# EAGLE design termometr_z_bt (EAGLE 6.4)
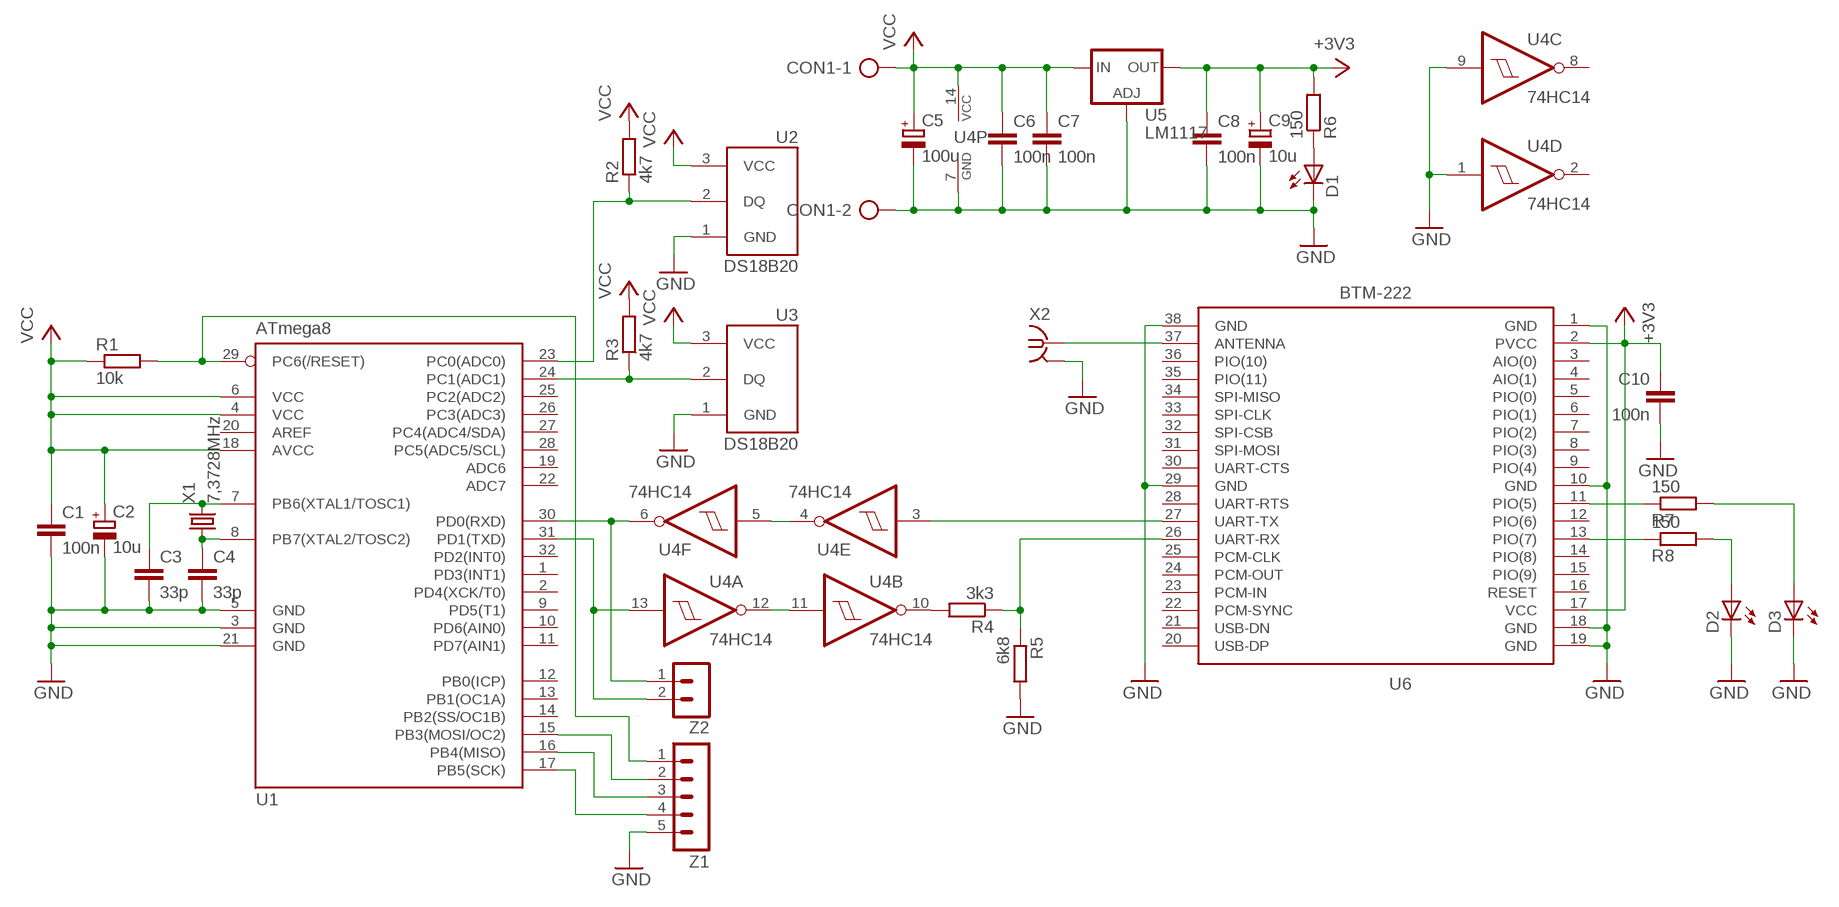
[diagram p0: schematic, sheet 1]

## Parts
C1  100n  C-EUC1206  [C1206]
C2  10u  CPOL-EUE2.5-5  [E2,5-5]
C3  33p  C-EUC1206  [C1206]
C4  33p  C-EUC1206  [C1206]
C5  100u  CPOL-EUE2.5-5  [E2,5-5]
C6  100n  C-EUC1206  [C1206]
C7  100n  C-EUC1206  [C1206]
C8  100n  C-EUC1206  [C1206]
C9  10u  CPOL-EUE2.5-5  [E2,5-5]
C10  100n  C-EUC1206  [C1206]
CON1  AK500/2  [AK500/2]
D1  LED5MM  [LED5MM]
D2  LED5MM  [LED5MM]
D3  LED5MM  [LED5MM]
R1  10k  R-EU_R1206  [R1206]
R2  4k7  R-EU_R1206  [R1206]
R3  4k7  R-EU_R1206  [R1206]
R4  3k3  R-EU_R1206  [R1206]
R5  6k8  R-EU_R1206  [R1206]
R6  150  R-EU_R1206  [R1206]
R7  150  R-EU_R1206  [R1206]
R8  150  R-EU_R1206  [R1206]
U1  ATmega8  MEGA8-AI  [TQFP32-08]
U2  DS18B20  [TO92-]
U3  DS18B20  [TO92-]
U4  74HC14  74HC14D  [SO14]
U5  LM1117  LD117AS50TR  [SOT223]
U6  BTM-222  BTM-222_ALL  [BTM-222]
X1  7,3728MHz  CRYSTALHC49S  [HC49/S]
X2  BU-SMA-G  [BU-SMA-G]
Z1  MA05-1  [MA05-1]
Z2  MA02-1  [MA02-1]

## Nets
+3V3: C8.1 C9.+ C10.1 R6.2 U5.4(OUT) U6.2(PVCC) U6.17(VCC)
GND: C1.2 C2.- C3.2 C4.2 C5.- C6.2 C7.2 C8.2 C9.- C10.2 CON1.2 D1.K(C) D2.K(C) D3.K(C) R5.2 U1.3(GND) U1.5(GND) U1.21(GND) U2.1(GND) U3.1(GND) U4.1(D:I) U4.7(P:GND) U4.9(C:I) U5.1(ADJ) U6.1(GND) U6.10(GND) U6.18(GND) U6.19(GND) U6.29(GND) U6.38(GND) X2.2(GND) Z1.5
N$1: D2.A R8.2
N$2: R7.1 U6.11(PIO(5))
N$3: D1.A R6.1
N$4: U4.3(E:I) U6.27(UART-TX)
N$5: R8.1 U6.13(PIO(7))
N$6: R1.2 U1.29(PC6(/RESET)) Z1.1
N$7: R2.1 U1.23(PC0(ADC0)) U2.2(DQ)
N$8: R3.1 U1.24(PC1(ADC1)) U3.2(DQ)
N$9: U4.11(B:I) U4.12(A:O)
N$10: U6.37(ANTENNA) X2.1
N$11: U4.4(E:O) U4.5(F:I)
N$12: U1.30(PD0(RXD)) U4.6(F:O) Z2.1
N$13: U1.31(PD1(TXD)) U4.13(A:I) Z2.2
N$14: R4.2 U4.10(B:O)
N$15: R4.1 R5.1 U6.26(UART-RX)
N$16: U1.15(PB3(MOSI/OC2)) Z1.2
N$17: U1.16(PB4(MISO)) Z1.3
N$18: U1.17(PB5(SCK)) Z1.4
N$19: D3.A R7.2
N$33: C3.1 U1.7(PB6(XTAL1/TOSC1)) X1.2
N$34: C4.1 U1.8(PB7(XTAL2/TOSC2)) X1.1
VCC: C1.1 C2.+ C5.+ C6.1 C7.1 CON1.1 R1.1 R2.2 R3.2 U1.4(VCC) U1.6(VCC) U1.18(AVCC) U2.3(VCC) U3.3(VCC) U4.14(P:VCC) U5.3(IN)
Unconnected: U1.1(PD3(INT1)) U1.2(PD4(XCK/T0)) U1.9(PD5(T1)) U1.10(PD6(AIN0)) U1.11(PD7(AIN1)) U1.12(PB0(ICP)) U1.13(PB1(OC1A)) U1.14(PB2(SS/OC1B)) U1.19(ADC6) U1.20(AREF) U1.22(ADC7) U1.25(PC2(ADC2)) U1.26(PC3(ADC3)) U1.27(PC4(ADC4/SDA)) U1.28(PC5(ADC5/SCL)) U1.32(PD2(INT0)) U4.2(D:O) U4.8(C:O) U6.3(AIO(0)) U6.4(AIO(1)) U6.5(PIO(0)) U6.6(PIO(1)) U6.7(PIO(2)) U6.8(PIO(3)) U6.9(PIO(4)) U6.12(PIO(6)) U6.14(PIO(8)) U6.15(PIO(9)) U6.16(RESET) U6.20(USB-DP) U6.21(USB-DN) U6.22(PCM-SYNC) U6.23(PCM-IN) U6.24(PCM-OUT) U6.25(PCM-CLK) U6.28(UART-RTS) U6.30(UART-CTS) U6.31(SPI-MOSI) U6.32(SPI-CSB) U6.33(SPI-CLK) U6.34(SPI-MISO) U6.35(PIO(11)) U6.36(PIO(10))

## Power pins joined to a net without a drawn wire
GND: X2.3(GND) X2.4(GND) X2.5(GND)

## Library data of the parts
C1 C3 C4 C6-C8 C10 = rcl:C-EU: CAPACITOR, European symbol
C2 C5 C9 = rcl:CPOL-EU: POLARIZED CAPACITOR, European symbol
CON1 = con-ptr500:AK500/2: CONNECTOR
D1-D3 = led:LED: LED
R1-R8 = rcl:R-EU_: RESISTOR, European symbol
U1 = atmel:MEGA8: MICROCONTROLLER 8 Kbytes FLASH, 1 kbytes SRAM, 512 bytes EEPROM, USART, 6-channel 10 bit ADC, 2-channel 8 bit ADC Pin compatible with Atmega48, ATMega88, ATMega168 Source: avr.lbr
U2 U3 = 1wire:DS18B20: Programmable Resolution Digital Thermometer This chip provides a onewire thermosensor with approx. 0.5°C accuracy. A programmable over/undertemperure alarm is available. The precision can be set from 9..12 bits. Notes: Vdd must be applied for accurate measurements at low temperatures, as the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
U4 = 74xx-eu:74*14: Hex schmitt trigger INVERTER
U5 = v-reg:LD117A?*: Low drop fixed and adjustable positive voltage regulators 1 A Source: http://www.st.com/stonline/products/literature/ds/7194/ld1117axx.pdf
U6 = bluetooth:BTM-222_ALL
X1 = crystal:CRYSTAL: CRYSTAL
X2 = con-coax:BU-SMA-G: FEMALE SMA CONNECTOR Radiall distributor RS 193-9117
Z1 = con-lstb:MA05-1: PIN HEADER
Z2 = con-lstb:MA02-1: PIN HEADER

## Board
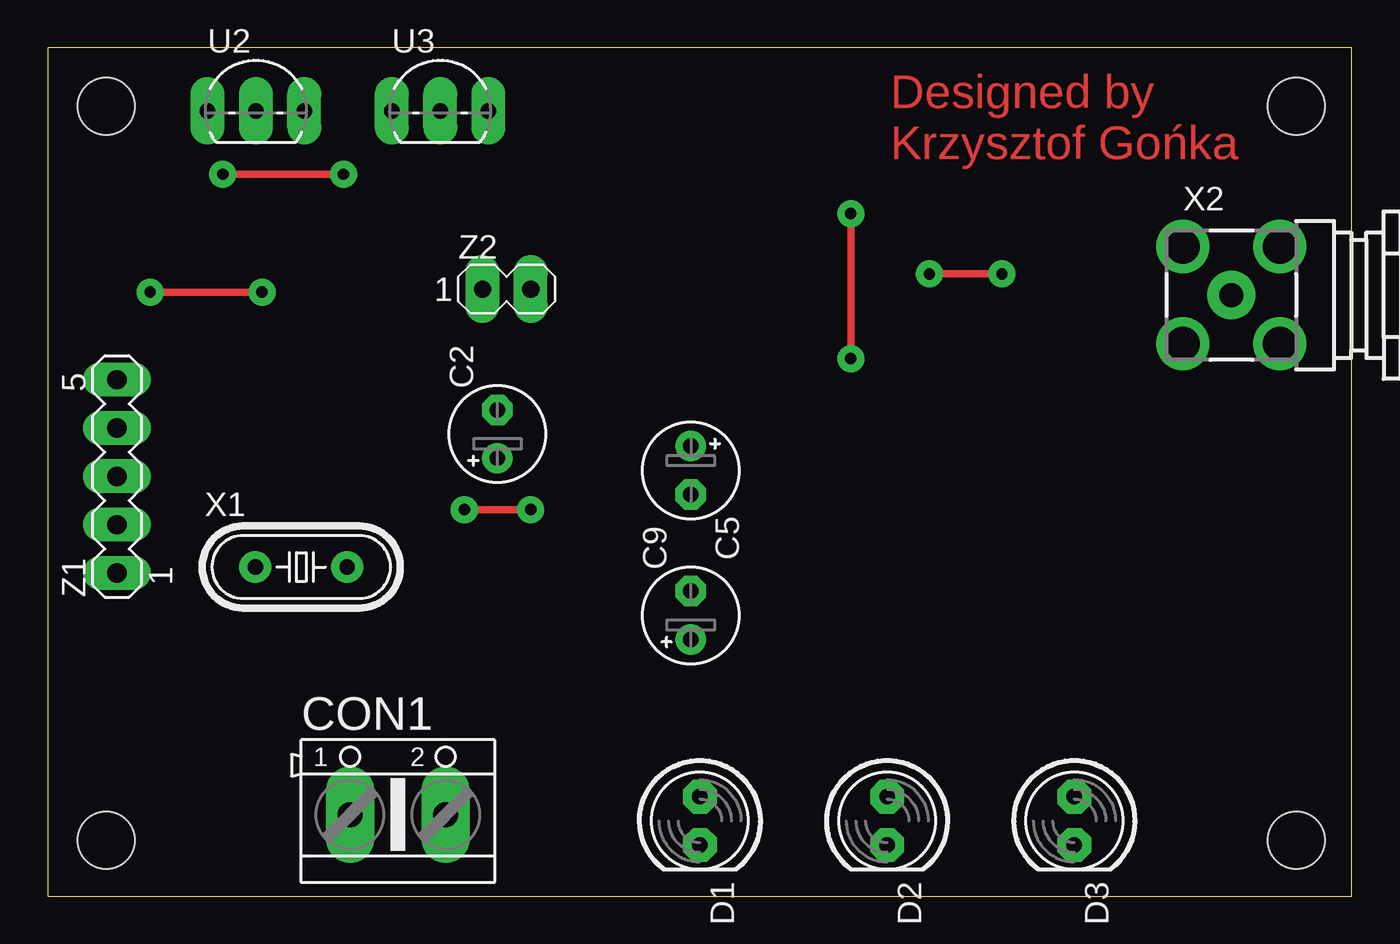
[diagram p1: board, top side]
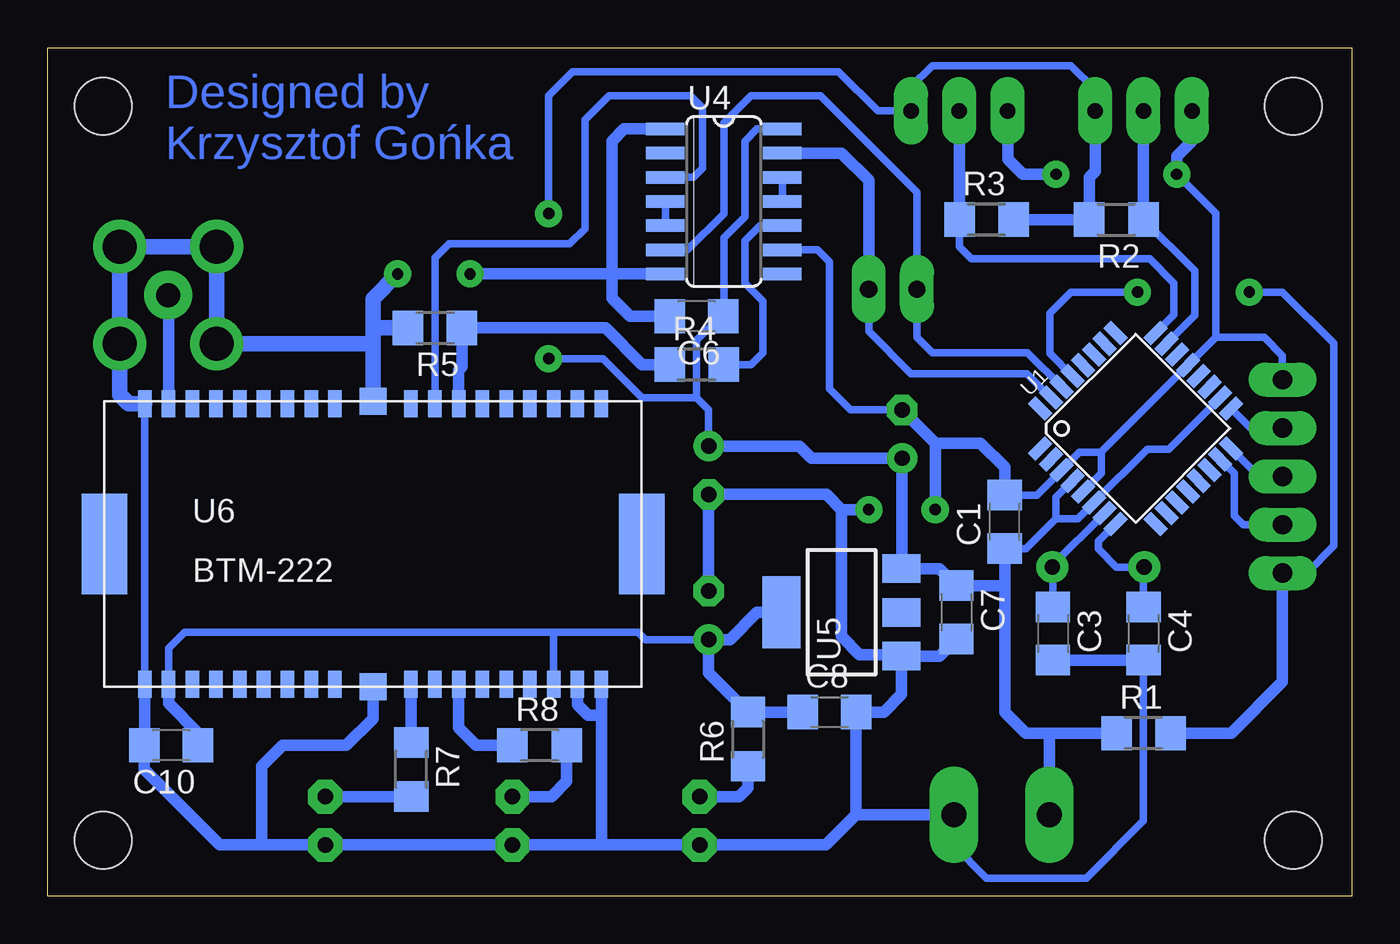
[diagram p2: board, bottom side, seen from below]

Size 68.57 x 44.6 mm. Coordinates in mm from the lower left corner, seen from the top.
Outline: 0,0 68.57,0 68.57,44.6 0,44.6 0,0
Copper layers (1*16): Top 0.035mm / dielectric 1.5mm / Bottom 0.035mm
Design rules "default": minimum track width 10mil, minimum drill 24mil, track to track 8mil, track to pad 8mil, pad to pad 8mil, via to via 8mil, smd to smd 8mil, copper to edge 40mil, drill to drill 8mil, minimum pad ring 10mil, minimum via ring 8mil, stop-mask expansion 4mil, vias tented up to drill 0mil, thermal gap 10mil
Holes 3 mm at 3.09,41.52 3.09,2.94 65.63,2.94 65.63,41.52

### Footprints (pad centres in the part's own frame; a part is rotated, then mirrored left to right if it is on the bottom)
C1206 = smd 1.6 x 1.8: 1 -1.4,0; 2 1.4,0
E2,5-5 = drill 0.813 pad 1.6: + -1.27,0 | drill 0.813 pad 1.6 octagon: - 1.27,0
AK500/2 = drill 1.321 pad 2.54 long: 1 -2.515,0; 2 2.515,0
LED5MM = drill 0.813 pad 1.778 octagon: A -1.27,0; K 1.27,0
R1206 = smd 1.6 x 1.803: 1 -1.422,0; 2 1.422,0
TQFP32-08 = smd 1.27 x 0.559: 1 -4.293,2.8; 2 -4.293,2; 3 -4.293,1.2; 4 -4.293,0.4; 5 -4.293,-0.4; 6 -4.293,-1.2; 7 -4.293,-2; 8 -4.293,-2.8; 17 4.293,-2.8; 18 4.293,-2; 19 4.293,-1.2; 20 4.293,-0.4; 21 4.293,0.4; 22 4.293,1.2; 23 4.293,2; 24 4.293,2.8 | smd 0.559 x 1.27: 9 -2.8,-4.293; 10 -2,-4.293; 11 -1.2,-4.293; 12 -0.4,-4.293; 13 0.4,-4.293; 14 1.2,-4.293; 15 2,-4.293; 16 2.8,-4.293; 25 2.8,4.293; 26 2,4.293; 27 1.2,4.293; 28 0.4,4.293; 29 -0.4,4.293; 30 -1.2,4.293; 31 -2,4.293; 32 -2.8,4.293
TO92- = drill 0.813 pad 1.778 long: 1 -2.54,0; 2 0,0; 3 2.54,0
SO14 = smd 0.66 x 2.032: 1 -3.81,-3.073; 2 -2.54,-3.073; 3 -1.27,-3.073; 4 0,-3.073; 5 1.27,-3.073; 6 2.54,-3.073; 7 3.81,-3.073; 8 3.81,3.073; 9 2.54,3.073; 10 1.27,3.073; 11 0,3.073; 12 -1.27,3.073; 13 -2.54,3.073; 14 -3.81,3.073
SOT223 = smd 1.5 x 2: 1 -2.3,-3.15; 2 0,-3.15; 3 2.3,-3.15 | smd 3.8 x 2: 4 0,3.15
BTM-222 = smd 0.711 x 1.422: 1 -12.5,-3.625; 2 -11.25,-3.625; 3 -10,-3.625; 4 -8.75,-3.625; 5 -7.5,-3.625; 6 -6.25,-3.625; 7 -5,-3.625; 8 -3.75,-3.625; 9 -2.5,-3.625; 11 1.5,-3.625; 12 2.75,-3.625; 13 4,-3.625; 14 5.25,-3.625; 15 6.5,-3.625; 16 7.75,-3.625; 17 9,-3.625; 18 10.25,-3.625; 19 11.5,-3.625; 20 11.5,11.125; 21 10.25,11.125; 22 9,11.125; 23 7.75,11.125; 24 6.5,11.125; 25 5.25,11.125; 26 4,11.125; 27 2.75,11.125; 28 1.5,11.125; 30 -2.5,11.125; 31 -3.75,11.125; 32 -5,11.125; 33 -6.25,11.125; 34 -7.5,11.125; 35 -8.75,11.125; 36 -10,11.125; 37 -11.25,11.125; 38 -12.5,11.125 | smd 1.422 x 1.4: 10 -0.5,-3.75; 29 -0.5,11.25 | smd 2.4 x 5.3: $AGND -14.625,3.75; $BGND 13.625,3.75
HC49/S = drill 0.813 pad 1.676: 1 -2.413,0; 2 2.413,0
BU-SMA-G = drill 1.27 pad 2.54: 1 0,0 | drill 1.778 pad 2.794: 2 -2.55,2.55; 3 2.55,2.55; 4 2.55,-2.55; 5 -2.55,-2.55
MA05-1 = drill 1.016 pad 1.778 long: 1 -5.08,0; 2 -2.54,0; 3 0,0; 4 2.54,0; 5 5.08,0
MA02-1 = drill 0.9 pad 1.778 long: 1 -2.54,0; 2 0,0

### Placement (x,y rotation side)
C1  18.26,19.68 90 bottom
C2  23.65,24.29 90 top
C3  15.72,13.81 270 bottom
C4  10.95,13.81 270 bottom
C5  33.81,22.38 270 top
C6  34.45,30.48 180 bottom
C7  20.8,14.92 270 bottom
C8  27.46,9.68 0 bottom
C9  33.81,14.76 90 top
C10  62.07,7.94 180 bottom
CON1  18.41,4.29 0 top
D1  34.29,3.97 270 top
D2  44.13,3.97 270 top
D3  53.98,3.97 270 top
R1  10.95,8.57 0 bottom
R2  12.38,35.56 180 bottom
R3  19.21,35.56 0 bottom
R4  34.45,27.94 0 bottom
R5  48.21,29.87 180 bottom
R6  31.75,8.26 90 bottom
R7  49.45,6.67 270 bottom
R8  42.7,7.94 0 bottom
U1  11.37,24.59 45 bottom
U2  10.95,41.27 0 top
U3  20.64,41.27 0 top
U4  33.02,36.51 270 bottom
U5  26.83,14.92 90 bottom
U6  50.96,14.76 0 bottom
X1  13.34,17.3 0 top
X2  62.23,31.59 0 top
Z1  3.65,22.07 90 top
Z2  25.4,31.91 0 top

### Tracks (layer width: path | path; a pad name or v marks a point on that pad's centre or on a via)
+3V3
  Bottom 0.406: 60.64,7.97 C10.1 | U6.17 41.96,13.83 41.91,13.88 | U6.2 62.21,13.04 61.37,13.88 41.91,13.88 | R6.2 | 41.91,13.88 37.53,13.88 37.15,13.49 C9.+
  Bottom 0.61: U6.2 62.21,10.14 60.64,8.57 60.64,7.97 | C8.1 R6.2 | U5.4 31.27,14.92 32.7,13.49 C9.+ 33.81,11.74 R6.2
GND  (via drill 0.6 pad 1.42)
  Top 0.406: v25.4,20.32 v21.91,20.32 | v46.35,32.7 v50.16,32.7 | v15.56,37.94 v9.21,37.94
  Bottom 0.406: U6.1 U6.38 | C10.2 63.5,7.91 | 51.43,29.87 51.46,29.84 | 51.47,29.04 51.46,29.05 | U4.9 28.1,33.97 27.46,33.34 27.46,26.67 26.35,25.56 C2.- | C1.2 16.57,21.09 U1.3 14.32,23.34 13.18,23.34 | CON1.2 20.95,4.26 20.95,2.7 19.21,0.95 13.97,0.95 10.95,3.97 C4.2 | 23.76,12.7 U5.1 | U1.5 13.18,22.22 13.18,23.34 | 13.18,23.34 13.18,23.35 U1.21 7.16,29.37 | 7.16,29.37 4.6,29.37 3.65,28.42 Z1.5 | 7.16,29.37 7.16,35.89 v9.21,37.94 | X2.4
  Bottom 0.61: U6.1 C10.2 | 57.31,2.7 D3.K D2.K 39.46,2.7 | 57.31,2.7 59.53,2.7 63.5,6.67 63.5,7.91 | U6.10 51.46,9.34 52.86,7.94 56.2,7.94 57.31,6.83 57.31,2.7 | U6.19 39.46,9.53 | U6.18 40.71,10.07 40.16,9.53 39.46,9.53 | C9.- C5.- 27.62,21.11 26.83,20.32 | C7.2 21.7,12.62 U5.1 23.68,10.61 24.61,9.68 C8.2 26.06,4.29 | U4.7 38.89,32.7 | 38.89,32.7 v46.35,32.7 | 38.89,32.7 38.89,39.69 38.26,40.32 U4.1 | C6.2 37.94,30.48 38.89,31.43 38.89,32.7 | v15.56,37.94 17.3,37.94 18.1,38.73 U3.1 | C3.2 C4.2 | 26.06,4.29 CON1.2 | 26.06,4.29 27.65,2.7 D1.K 39.46,2.7 | 39.46,9.53 39.46,2.7 | 26.83,20.32 26.83,13.65 25.88,12.7 23.76,12.7 | v9.21,37.94 9.21,38.89 8.41,39.69 U2.1 | v25.4,20.32 26.83,20.32 | v21.91,20.32 21.91,23.81 | 21.91,23.81 C2.- | C1.2 18.26,22.54 19.53,23.81 21.91,23.81
  Bottom 0.813: X2.4 X2.3 X2.2 X2.5 51.47,29.04 | U6.29 51.46,29.05 51.46,29.84 51.46,31.41 v50.16,32.7 | R5.2 51.43,29.87 | U6.38 64.31,25.89 64.77,26.35 X2.4
N$1
  Bottom 0.406: R8.2
  Bottom 0.61: D2.A 42.07,5.24 41.27,6.03 R8.2
N$2
  Bottom 0.406: R7.1
  Bottom 0.61: U6.11 R7.1
N$3
  Bottom 0.61: D1.A 32.23,5.24 31.75,5.71 R6.1
N$4
  Bottom 0.406: U4.3 34.61,37.78 34.13,38.26 34.13,41.43 34.77,42.07 39.05,42.07 40.32,40.8 40.32,35.08 41.12,34.29 47.47,34.29 48.21,33.55 U6.27
N$5
  Bottom 0.61: U6.13 46.96,8.86 46.04,7.94 R8.1
N$6  (via drill 0.6 pad 1.42)
  Top 0.406: v5.4,31.75 v11.27,31.75
  Bottom 0.406: Z1.1 2.38,16.99 0.95,18.41 0.95,29.05 3.65,31.75 v5.4,31.75 | U1.29 15.88,28.52 15.88,30.64 14.76,31.75 v11.27,31.75
  Bottom 0.61: Z1.1 3.65,11.27 6.35,8.57 R1.2
N$7
  Bottom 0.406: R2.1 8.26,32.86 8.26,30.53 U1.23
  Bottom 0.61: U2.2 R2.1
N$8
  Bottom 0.406: R3.1 20.64,34.13 20,33.5 10.64,33.5 9.37,32.23 9.37,30.55 U1.24
  Bottom 0.61: U3.2 R3.1
N$9
  Bottom 0.406: U4.12 U4.11
N$10
  Bottom 0.61: U6.37 62.21,31.57 X2.1
N$11
  Bottom 0.406: U4.4 U4.5
N$12
  Bottom 0.406: U4.6 34.92,33.97 33.02,35.88 33.02,40.64 31.59,42.07 27.94,42.07 22.86,36.99 Z2.1 22.86,29.37 22.07,28.57 17.06,28.57 U1.30
N$13
  Bottom 0.406: U1.31 17.08,27.46 23.18,27.46 25.4,29.69 Z2.2
  Bottom 0.61: U4.13 26.83,39.05 25.4,37.62 Z2.2
N$14
  Bottom 0.406: U4.10 31.11,35.24 31.91,34.45 31.91,32.23 30.96,31.27 30.96,28.57 31.59,27.94 R4.2
N$15
  Bottom 0.61: U6.26 46.96,27.65 46.78,27.83 R5.1 39.24,29.87 37.31,27.94 R4.1
N$16
  Bottom 0.406: Z1.2 5.71,19.53 6.19,20 6.19,22.23 U1.15
N$17
  Bottom 0.406: Z1.3 4.89,22.07 U1.16
N$18
  Bottom 0.406: Z1.4 5.32,24.61 U1.17
N$19
  Bottom 0.406: R7.2
  Bottom 0.61: D3.A R7.2
N$33
  Bottom 0.406: U1.7 15.75,17.38 X1.2 15.72,17.27 C3.1
N$34
  Bottom 0.406: C4.1 10.95,17.27 X1.1 12.38,17.3 13.34,18.26 13.34,18.66 U1.8
VCC  (via drill 0.6 pad 1.42)
  Top 0.406: v42.23,28.26 v42.23,35.88
  Bottom 0.406: U4.14 31.27,40.32 31.91,39.69 31.91,35.72 33.02,34.61 33.02,30.51 C6.1 33.18,30.48 34.45,29.21 34.45,26.19 | v42.23,28.26 39.37,28.26 37.31,26.19 34.45,26.19 | v42.23,35.88 42.23,42.07 40.96,43.34 26.99,43.34 24.92,41.27 U3.3 23.18,42.55 22.07,43.66 14.76,43.66 13.49,42.39 U2.3 | C5.+ 33.81,25.56 34.45,26.19 | R2.2 | U1.4 15.56,20.97 15.56,19.84 | 15.56,19.84 14.42,19.84 U1.6 10.77,23.5 9.64,23.5 U1.18 | 15.56,19.84 17.14,18.26 18.23,18.26 C1.1 | 18.29,16.32 18.26,16.35 | 15.9,8.55 15.88,8.57 | 23.65,17.25 U5.3
  Bottom 0.61: U5.3 21.7,17.22 C7.1 18.29,16.32 | U2.3 13.49,38.1 13.81,37.78 R2.2 | R3.2 R2.2 | C1.1 18.26,16.35 18.26,9.68 17.14,8.57 15.88,8.57 R1.1 | CON1.1 15.9,8.55 | 23.65,17.25 C2.+ 28.42,23.02 29.05,23.65 C5.+

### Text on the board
Top: Designed by / Krzysztof Gońka
Bottom: Designed by / Krzysztof Gońka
